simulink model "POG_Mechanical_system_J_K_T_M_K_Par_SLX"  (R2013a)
settings: Solver=ode45  StartTime=0.0  StopTime=10.0  MaxStep=0.001  RelTol=1e-3
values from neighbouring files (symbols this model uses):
  b_1 = 1*Nm/(10*rpm)    (= 0.954929658551)    [POG_Mechanical_system_J_K_T_M_K_Par_SLX_m.m]    (also in POG_Mechanical_system_J_K_T_M_K_SLX_m.m = 1; POG_Mechanical_system_J_K_T_M_K_SuperBlock_SLX_m.m = 1; POG_Mechanical_system_J_K_T_M_K_NL_SLX_m.m)
  b_2 = 50*Newton/(2*meters/sec)    (= 25)    [POG_Mechanical_system_J_K_T_M_K_Par_SLX_m.m]    (also in POG_Mechanical_system_J_K_T_M_K_SLX_m.m = 1; POG_Mechanical_system_J_K_T_M_K_SuperBlock_SLX_m.m = 1; POG_Mass_Linear_Control_SLX_m.m; POG_Mechanical_system_J_K_T_M_K_NL_SLX_m.m)
  J = 1*kg*(30*cm)^2    (= 0.09)    [POG_Mechanical_system_J_K_T_M_K_Par_SLX_m.m]    (also in POG_Mechanical_system_J_K_T_M_K_SLX_m.m = 1; POG_Mechanical_system_J_K_T_M_K_SuperBlock_SLX_m.m = 1; POG_Mechanical_system_J_K_T_M_K_NL_SLX_m.m)
  K_1 = 5*Newton/(1*mm)    (= 5000)    [POG_Mechanical_system_J_K_T_M_K_Par_SLX_m.m]    (also in POG_Mechanical_system_J_K_T_M_K_SLX_m.m = 1; POG_Mechanical_system_J_K_T_M_K_SuperBlock_SLX_m.m = 1; POG_Mechanical_system_J_K_T_M_K_NL_SLX_m.m)
  K_2 = 20*Newton/(1*cm)    (= 2000)    [POG_Mechanical_system_J_K_T_M_K_Par_SLX_m.m]    (also in POG_Mechanical_system_J_K_T_M_K_SLX_m.m = 1; POG_Mechanical_system_J_K_T_M_K_SuperBlock_SLX_m.m = 1; POG_Mechanical_system_J_K_T_M_K_NL_SLX_m.m)
  M = 10*kg    (= 10)    [POG_Mechanical_system_J_K_T_M_K_Par_SLX_m.m]    (also in POG_Mechanical_system_J_K_T_M_K_SLX_m.m = 1; POG_Mechanical_system_J_K_T_M_K_SuperBlock_SLX_m.m = 1; POG_Mass_Linear_Control_SLX_m.m; POG_Mechanical_system_J_K_T_M_K_NL_SLX_m.m)
  P_2_0 = 0    [POG_Mechanical_system_J_K_T_M_K_Par_SLX_m.m]    (also in POG_Mechanical_system_J_K_T_M_K_SLX_m.m; POG_Mechanical_system_J_K_T_M_K_SuperBlock_SLX_m.m; POG_Mechanical_system_J_K_T_M_K_NL_SLX_m.m)
  P_7_0 = 0    [POG_Mechanical_system_J_K_T_M_K_Par_SLX_m.m]    (also in POG_Mechanical_system_J_K_T_M_K_SLX_m.m; POG_Mechanical_system_J_K_T_M_K_SuperBlock_SLX_m.m)
  R = 40*cm    (= 0.4)    [POG_Mechanical_system_J_K_T_M_K_Par_SLX_m.m]    (also in POG_Mechanical_system_J_K_T_M_K_SLX_m.m = 1; POG_Mechanical_system_J_K_T_M_K_SuperBlock_SLX_m.m = 1; POG_Mechanical_system_J_K_T_M_K_NL_SLX_m.m)
  T = 10*Nm    (= 10)    [POG_Mechanical_system_J_K_T_M_K_Par_SLX_m.m]    (also in POG_Mechanical_system_J_K_T_M_K_SLX_m.m; POG_Mechanical_system_J_K_T_M_K_SuperBlock_SLX_m.m; POG_Mechanical_system_J_K_T_M_K_NL_SLX_m.m = 2)
  Ts = Tfin/Nr_Ts_Points    (= 0.0025)    [POG_Mechanical_system_J_K_T_M_K_Par_SLX_m.m]    (also in POG_Mechanical_system_J_K_T_M_K_SLX_m.m = 0.005; POG_Mechanical_system_J_K_T_M_K_SuperBlock_SLX_m.m = 0.005; POG_Mass_Linear_Control_SLX_m.m; POG_Mechanical_system_J_K_T_M_K_NL_SLX_m.m)
  v_d = 0    [POG_Mechanical_system_J_K_T_M_K_Par_SLX_m.m]    (also in POG_Mechanical_system_J_K_T_M_K_SLX_m.m; POG_Mechanical_system_J_K_T_M_K_SuperBlock_SLX_m.m; POG_Mechanical_system_J_K_T_M_K_NL_SLX_m.m)
  x_6_0 = 0    [POG_Mechanical_system_J_K_T_M_K_Par_SLX_m.m]    (also in POG_Mechanical_system_J_K_T_M_K_SLX_m.m; POG_Mechanical_system_J_K_T_M_K_SuperBlock_SLX_m.m; POG_Mechanical_system_J_K_T_M_K_NL_SLX_m.m)
  x_9_0 = 0    [POG_Mechanical_system_J_K_T_M_K_Par_SLX_m.m]    (also in POG_Mechanical_system_J_K_T_M_K_SLX_m.m; POG_Mechanical_system_J_K_T_M_K_SuperBlock_SLX_m.m; POG_Mechanical_system_J_K_T_M_K_NL_SLX_m.m)

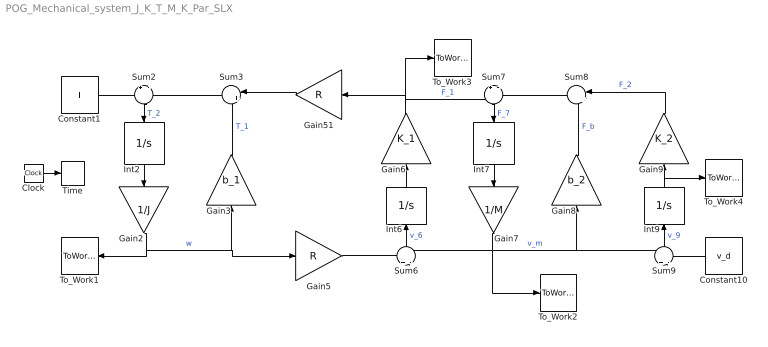
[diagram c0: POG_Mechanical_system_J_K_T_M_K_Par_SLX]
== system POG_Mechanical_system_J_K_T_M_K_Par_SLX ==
  Clock : Clock
  Constant1 : Constant  Value=T
  Constant10 : Constant  Value=v_d
  Gain2 : Gain  Gain=1/J
  Gain3 : Gain  Gain=b_1
  Gain5 : Gain  Gain=R
  Gain51 : Gain  Gain=R
  Gain6 : Gain  Gain=K_1
  Gain7 : Gain  Gain=1/M
  Gain8 : Gain  Gain=b_2
  Gain9 : Gain  Gain=K_2
  Int2 : Integrator  InitialCondition=P_2_0
  Int6 : Integrator  InitialCondition=x_6_0
  Int7 : Integrator  InitialCondition=P_7_0
  Int9 : Integrator  InitialCondition=x_9_0
  Sum{2,6..7,9} (4 alike) : Sum  Inputs=+|-
  Sum3 : Sum  Inputs=|++
  Sum8 : Sum  Inputs=|++
  Time : ToWorkspace  VariableName=t  SampleTime=Ts
  To_Work1 : ToWorkspace  VariableName=w_1  SampleTime=Ts
  To_Work2 : ToWorkspace  VariableName=w_m  SampleTime=Ts
  To_Work3 : ToWorkspace  VariableName=F_1  SampleTime=Ts
  To_Work4 : ToWorkspace  VariableName=x  SampleTime=Ts
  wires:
  Constant1/1 -> Sum2/1
  Sum3/1 -> Sum2/2
  Gain2/1 -> To_Work1/1, Gain3/1, Gain5/1  "w"
  Sum2/1 -> Int2/1  "T_2"
  Int2/1 -> Gain2/1
  Gain51/1 -> Sum3/1
  Gain3/1 -> Sum3/2  "T_1"
  Gain5/1 -> Sum6/1
  Gain6/1 -> To_Work3/1, Gain51/1, Sum7/1  "F_1"
  Gain7/1 -> To_Work2/1, Sum6/2, Gain8/1, Sum9/1  "v_m"
  Sum6/1 -> Int6/1  "v_6"
  Int6/1 -> Gain6/1
  Sum8/1 -> Sum7/2
  Sum7/1 -> Int7/1  "F_7"
  Int7/1 -> Gain7/1
  Gain9/1 -> Sum8/1  "F_2"
  Gain8/1 -> Sum8/2  "F_b"
  Constant10/1 -> Sum9/2
  Sum9/1 -> Int9/1  "v_9"
  Int9/1 -> To_Work4/1, Gain9/1
  Clock/1 -> Time/1
